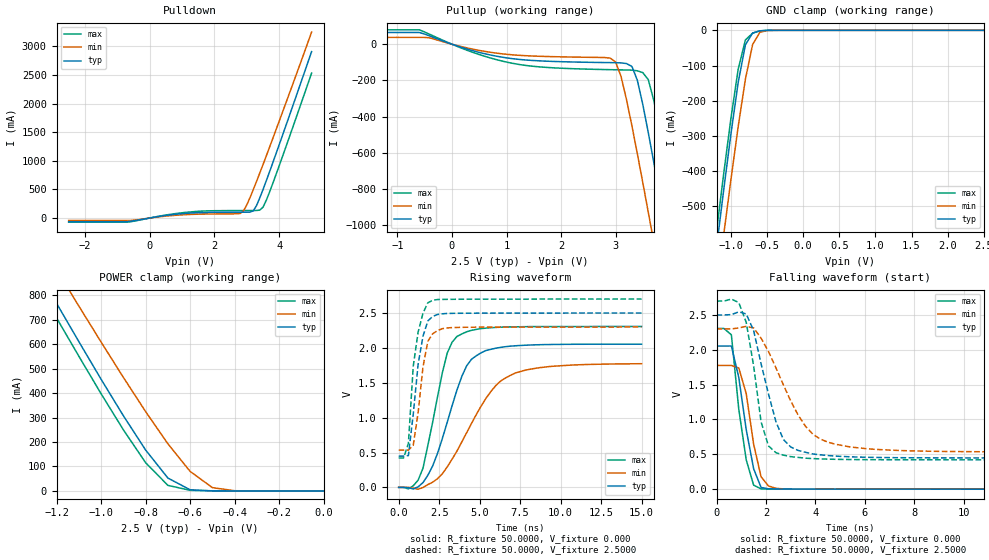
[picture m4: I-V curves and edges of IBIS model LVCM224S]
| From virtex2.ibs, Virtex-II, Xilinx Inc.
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|   Model LVCM224S
[Model]   LVCM224S
Model_type   I/O
Polarity   Non-Inverting
Enable   Active-Low
Vinh = 1.7V
Vinl = 0.7V
Vmeas =   1.2500V
Cref =  0pF
Rref =   1.0000M
Vref =  0.000V
C_comp   7.0000pF   6.0000pF   8.0000pF
[Temperature Range]   25.0000   100.0000   0.000
[Voltage Range]   2.5000V   2.3000V   2.7000V
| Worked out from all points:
|   slope of the pulldown table from 0 to 0.375 V, typ, clamps not added: 10.7 ohm
|   slope of the pullup table from 0 to 0.375 V, typ, clamps not added: 10.6 ohm
|   GND clamp passes 1 mA (typ) near -0.57 V on its own axis
|   POWER clamp passes 1 mA (typ) near -0.52 V on its own axis
|   rising waveform, R_fixture 50.0000, V_fixture 0.000: 20-80 % time 1.73ns typ, 2.69ns min, 1.24ns max; typ from 0 V to 2.05 V
|   rising waveform, R_fixture 50.0000, V_fixture 2.5000: 20-80 % time 640ps typ, 597ps min, 555ps max; typ from 0.448 V to 2.5 V
|   falling waveform, R_fixture 50.0000, V_fixture 0.000: 20-80 % time 564ps typ, 526ps min, 479ps max; typ from 2.05 V to 0 V
|   falling waveform, R_fixture 50.0000, V_fixture 2.5000: 20-80 % time 913ps typ, 1.5ns min, 605ps max; typ from 2.5 V to 0.448 V
[Pulldown]
| voltage   I(typ)   I(min)   I(max)
-2.5V     -63.55mA   -42.86mA   -72.65mA
-700mV    -63.55mA   -42.86mA   -72.65mA
1.1V      80.91mA    58.77mA    98.16mA
2.8V      102.3mA    80.57mA    130.8mA
2.9V      102.4mA    128mA      131mA
3V        102.7mA    231.1mA    131.2mA
3.2V      125.9mA    497mA      131.6mA
3.4V      351.8mA    787.1mA    138.6mA
3.5V      497.9mA    935.8mA    190.1mA
3.7V      806.1mA    1.237A     451.4mA
4V        1.283A     1.695A     914.8mA
5V        2.91A      3.252A     2.535A
[Pullup]
| voltage   I(typ)   I(min)   I(max)
-2.5V     64.88mA    37.65mA    79.8mA
-600mV    64.88mA    37.65mA    79.8mA
1V        -75.49mA   -55.69mA   -98.73mA
2.9V      -101.8mA   -76.75mA   -140.8mA
3V        -102.3mA   -97.7mA    -141.4mA
3.2V      -107mA     -305.7mA   -142.5mA
3.4V      -200.1mA   -607.2mA   -147.1mA
3.6V      -489.3mA   -930mA     -196.2mA
3.7V      -652.2mA   -1.094A    -310mA
4V        -1.16A     -1.597A    -786.4mA
4.2V      -1.506A    -1.935A    -1.127A
5V        -2.913A    -3.304A    -2.527A
[GND_clamp]
| voltage   I(typ)   I(min)   I(max)
-2.5V     -2.881A    -2.936A    -2.838A
-1.2V     -617mA     -740.6mA   -570.6mA
-1.1V     -452.1mA   -579.7mA   -406.1mA
-1V       -293.4mA   -423mA     -249mA
-900mV    -148mA     -273.4mA   -110.1mA
-800mV    -41mA      -138.5mA   -27.22mA
-700mV    -7.569mA   -40.19mA   -8.128mA
-600mV    -1.403mA   -5.589mA   -1.597mA
-500mV    -127.6uA   -662.5uA   -122uA
2.5V      397.5nA    2.548uA    351.3nA
[POWER_clamp]
| voltage   I(typ)   I(min)   I(max)
-2.5V     2.874A     2.908A     2.816A
-1.3V     925.8mA    1.055A     866.1mA
-1.2V     767.5mA    905.5mA    707.7mA
-1.1V     610.9mA    756.3mA    551.2mA
-1V       456.9mA    609.1mA    397.6mA
-900mV    307.7mA    464.5mA    250.2mA
-800mV    167.5mA    324.6mA    115.6mA
-700mV    52.75mA    192.9mA    22.81mA
-600mV    4.571mA    79.88mA    2.444mA
-500mV    271.3uA    13.45mA    251.8uA
-400mV    16.93uA    820.9uA    15.04uA
0V        397.5nA    368nA      428.7nA
[Ramp]
| variable   typ   min   max
dV/dt_r   1.2318/1.7155n   1.0638/2.6796n   1.3842/1.2381n
dV/dt_f   1.2313/0.9134n   1.0596/1.4895n   1.3672/0.6487n
R_load = 50.0000
[Rising Waveform]
R_fixture = 50.0000
V_fixture = 0.000
| time   V(typ)   V(min)   V(max)
0s        3.831uV    4.714uV    3.644uV
900ps     -22.64mV   -11.53mV   22.71mV
1.5ns     68.03mV    -1.937mV   273.7mV
2.1ns     308.1mV    74.15mV    937.8mV
3ns       935.4mV    294.5mV    1.927V
3.6ns     1.397V     521mV      2.164V
4.5ns     1.837V     918mV      2.252V
6ns       1.996V     1.46V      2.293V
7.2ns     2.03V      1.64V      2.303V
15ns      2.053V     1.773V     2.307V
[Rising Waveform]
R_fixture = 50.0000
V_fixture = 2.5000
V_fixture_min = 2.3000
V_fixture_max = 2.7000
| time   V(typ)   V(min)   V(max)
0s        447.9mV    533.7mV    421.4mV
300ps     447.9mV    533.7mV    421.5mV
600ps     456.1mV    533.6mV    630.9mV
900ps     1.05V      603.5mV    1.737V
1.2ns     1.764V     1.069V     2.225V
1.5ns     2.166V     1.726V     2.496V
1.8ns     2.386V     2.095V     2.647V
2.1ns     2.451V     2.203V     2.682V
3ns       2.494V     2.287V     2.696V
15ns      2.5V       2.3V       2.7V
[Falling Waveform]
R_fixture = 50.0000
V_fixture = 0.000
| time   V(typ)   V(min)   V(max)
0s        2.054V     1.776V     2.307V
300ps     2.054V     1.776V     2.307V
600ps     2.054V     1.776V     2.216V
900ps     1.603V     1.738V     1.145V
1.2ns     854.5mV    1.372V     420.7mV
1.5ns     292.9mV    645.6mV    57.54mV
1.8ns     24.45mV    177.4mV    3.551mV
2.1ns     4.799mV    45.54mV    1.808mV
2.7ns     1.67mV     3.968mV    1.367mV
15ns      12.85uV    -26.84uV   -24.02uV
[Falling Waveform]
R_fixture = 50.0000
V_fixture = 2.5000
V_fixture_min = 2.3000
V_fixture_max = 2.7000
| time   V(typ)   V(min)   V(max)
0s        2.5V       2.3V       2.7V
900ps     2.545V     2.314V     2.678V
1.2ns     2.515V     2.337V     2.395V
1.8ns     1.8V       2.168V     966.8mV
2.1ns     1.365V     1.976V     620.3mV
2.4ns     970.4mV    1.742V     524.1mV
2.7ns     713.9mV    1.498V     488.6mV
3.6ns     528.7mV    900.4mV    444.6mV
4.8ns     474.6mV    645.5mV    428.6mV
15ns      447.9mV    534mV      421.4mV
